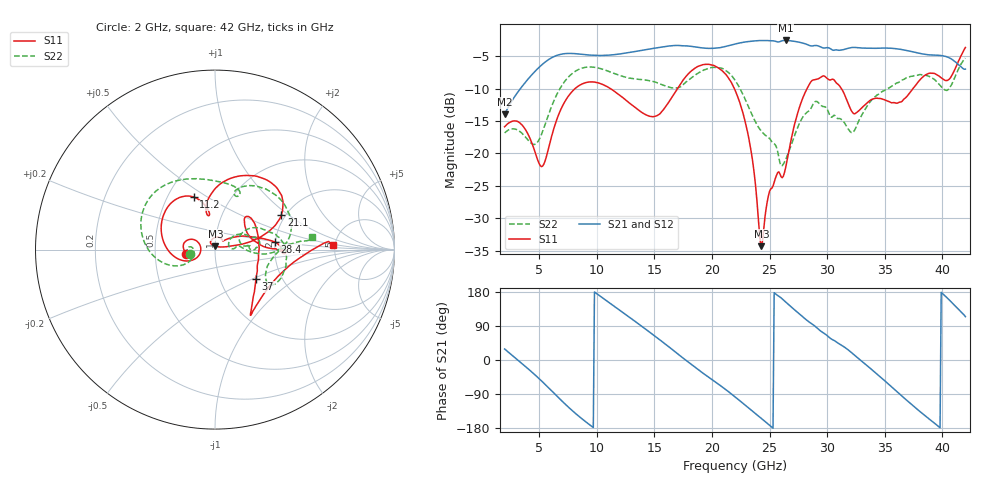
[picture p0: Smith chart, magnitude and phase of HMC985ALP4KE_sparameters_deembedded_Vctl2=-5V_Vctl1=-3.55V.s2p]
!s2p File: Measurements: S11, S21, S12, S22
# GHz S dB R 50.0
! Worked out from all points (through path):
!   401 points, 2 GHz to 42 GHz, reference 50 ohm
!   highest |S21| = -2.56 dB at 26.4 GHz (marker M1); lowest = -14.0 dB at 2 GHz (marker M2)
!   lowest |S11| = -34.3 dB at 24.3 GHz (marker M3), VSWR 1.04, Z = 50.2 + j1.91 ohm
!   |S11| at or under -10 dB: start of sweep to 8.113 GHz; 21.95 GHz to 28.25 GHz (6.308 GHz wide, 25.1 % of centre); 31.24 GHz to 37.45 GHz (6.211 GHz wide, 18.1 % of centre)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
!   |S22| runs from -21.9 to -5.3 dB; largest |S21 - S12| = 0.00061
!   S11 on the Smith chart (normalised r, x): 2 GHz: 0.73, -0.03; 11.2 GHz: 0.67, +0.44; 21.1 GHz: 1.90, +0.88; 28.4 GHz: 1.98, +0.19; 37 GHz: 1.48, -0.52; 42 GHz: 4.78, +0.43
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2  -15.90 -172.1  -13.99 29.1  -13.99 29.1  -16.84 -169.9
3.5  -15.59 162.4  -9.70 -9.3  -9.70 -9.3  -16.89 173.7
5.3  -21.96 -175.9  -6.22 -58.0  -6.22 -58.0  -16.61 -156.6
6.9  -13.14 -167.8  -4.69 -106.0  -4.69 -106.0  -9.71 -170.7
8.7  -9.30 147.9  -4.70 -154.8  -4.70 -154.8  -6.85 152.5
11.2  -10.02 112.0  -4.81 148.7  -4.81 148.7  -7.45 112.1
13.5  -13.14 99.6  -4.22 98.1  -4.22 98.1  -8.54 80.8
15.4  -14.00 102.7  -3.66 54.8  -3.66 54.9  -9.20 66.3
17.9  -7.80 77.5  -3.42 -4.6  -3.42 -4.6  -8.79 69.2
21.1  -7.62 27.4  -3.52 -75.8  -3.52 -75.8  -7.10 15.6
22  -10.20 18.3  -3.12 -97.2  -3.12 -97.2  -8.69 1.3
23.3  -18.66 11.8  -2.71 -129.4  -2.71 -129.4  -13.34 -4.7
24.3  -34.33 82.6  -2.58 -154.5  -2.58 -154.5  -16.60 5.2
25  -25.86 119.5  -2.61 -172.3  -2.61 -172.2  -17.70 8.1
26.4  -22.18 43.6  -2.56 153.0  -2.57 153.0  -20.95 29.7
28.4  -9.50 7.4  -3.29 101.0  -3.29 101.0  -13.46 18.8
28.7  -8.74 2.3  -3.42 95.0  -3.42 95.0  -12.66 17.2
32.4  -13.88 28.6  -3.64 12.0  -3.64 12.0  -16.36 26.3
35.4  -12.02 15.5  -3.76 -65.7  -3.75 -65.6  -9.87 17.6
37  -11.03 -35.5  -4.15 -108.7  -4.16 -108.7  -8.28 4.0
39.7  -8.05 -56.3  -4.86 -176.4  -4.86 -176.3  -9.30 -32.4
42  -3.65 2.2  -6.99 114.4  -6.99 114.5  -5.29 7.3
